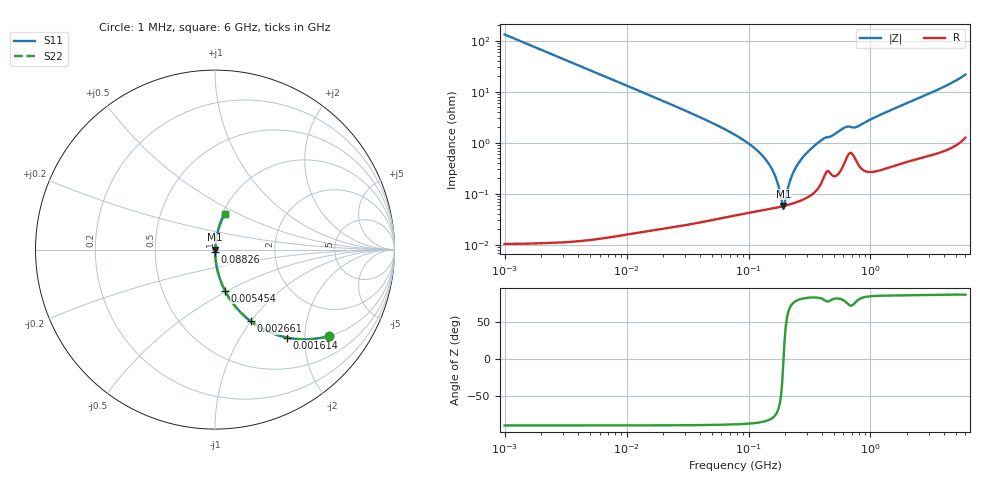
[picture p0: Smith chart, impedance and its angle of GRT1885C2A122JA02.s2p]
!Murata Part Number: GRT1885C2A122JA02
!These Parameters are Measured in Series Mode Connection
!Data Generated on Jun 19, 2026
!  o--ll--o
!Port1  Port2
!  o------o
!Operation Temp=25[degC], DC Bias Voltage=0[V]
!Freq. Start=1000[kHz] Stop=6[GHz] 401[Steps]
# Hz S RI R 50
!Freq.(Hz) S11(Real) S11(Imag) S21(Real) S21(Imag) S12(Real) S12(Imag) S22(Real) S22(Imag)
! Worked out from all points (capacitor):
!   401 points, 1 MHz to 6 GHz, reference 50 ohm
!   read as one part in series: C = 1.2 nF near 1.044 MHz
!   lowest |Z| = 57.1 mohm at 193.1 MHz (marker M1)
!   series resonance near 193.7 MHz, so ESL is about 560 pH
!   S11 on the Smith chart (normalised r, x): 1 MHz: 1.00, -2.64; 1.614 MHz: 1.00, -1.64; 2.661 MHz: 1.00, -0.99; 5.454 MHz: 1.00, -0.48; 88.26 MHz: 1.00, -0.02; 6 GHz: 1.02, +0.43
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1000000  0.6359 -0.4811  0.3641 0.4811  0.3641 0.4811  0.6359 -0.4811
1613609  0.4015 -0.4901  0.5985 0.4901  0.5985 0.4901  0.4015 -0.4901
2660982  0.1978 -0.3983  0.8022 0.3983  0.8022 0.3983  0.1978 -0.3983
4293785  0.0865 -0.281  0.9135 0.281  0.9135 0.281  0.0865 -0.281
5454306  0.0555 -0.2286  0.9445 0.2286  0.9445 0.2286  0.0555 -0.2286
1.843659e7  0.0052 -0.0706  0.9948 0.0706  0.9948 0.0706  0.0052 -0.0706
7.745967e7  0.000575 -0.0142  0.9994 0.0142  0.9994 0.0142  0.000575 -0.0142
8.825674e7  0.000534 -0.0118  0.9995 0.0118  0.9995 0.0118  0.000534 -0.0118
1.196694e8  0.000497 -0.00677  0.9995 0.00677  0.9995 0.00677  0.000497 -0.00677
1.455431e8  0.000508 -0.00393  0.9995 0.00393  0.9995 0.00393  0.000508 -0.00393
1.658303e8  0.000529 -0.00212  0.9995 0.00212  0.9995 0.00212  0.000529 -0.00212
1.848803e8  0.000556 -0.000634  0.9994 0.000634  0.9994 0.000634  0.000556 -0.000634
1.930997e8  0.000569 -4.35e-05  0.9994 4.35e-05  0.9994 4.35e-05  0.000569 -4.35e-05
2.016844e8  0.000585 0.000548  0.9994 -0.000548  0.9994 -0.000548  0.000585 0.000548
2.200158e8  0.000622 0.00174  0.9994 -0.00174  0.9994 -0.00174  0.000622 0.00174
2.400133e8  0.000669 0.00295  0.9993 -0.00295  0.9993 -0.00295  0.000669 0.00295
2.734687e8  0.000767 0.00482  0.9992 -0.00482  0.9992 -0.00482  0.000767 0.00482
3.325952e8  0.00103 0.00789  0.999 -0.00789  0.999 -0.00789  0.00103 0.00789
6.11486e8  0.00433 0.0191  0.9957 -0.0191  0.9957 -0.0191  0.00433 0.0191
7.767579e8  0.00444 0.02  0.9956 -0.02  0.9956 -0.02  0.00444 0.02
1.428092e9  0.005 0.0417  0.995 -0.0417  0.995 -0.0417  0.005 0.0417
6e9  0.0551 0.201  0.9449 -0.201  0.9449 -0.201  0.0551 0.201
